FUNCTION_BLOCK "Mult_1"
VERSION : 0.1

BEGIN
NETWORK
TITLE =
END_FUNCTION_BLOCK

FUNCTION_BLOCK "Mult_2"
VERSION : 0.1

BEGIN
NETWORK
TITLE =
END_FUNCTION_BLOCK

FUNCTION "Mult_3" : Void
VERSION : 0.1

BEGIN
NETWORK
TITLE =
END_FUNCTION

